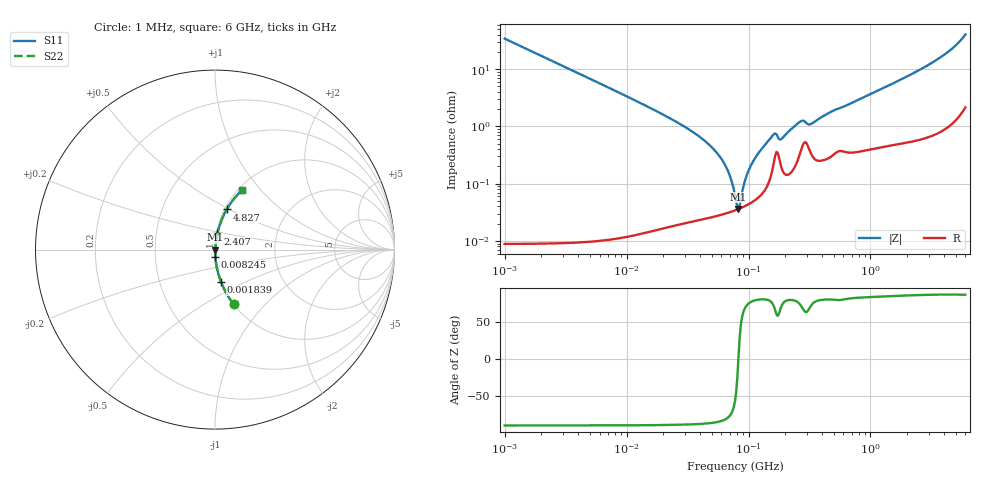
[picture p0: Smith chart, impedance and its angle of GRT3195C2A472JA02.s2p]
!Murata Part Number: GRT3195C2A472JA02
!These Parameters are Measured in Series Mode Connection
!Data Generated on Jun 19, 2026
!  o--ll--o
!Port1  Port2
!  o------o
!Operation Temp=25[degC], DC Bias Voltage=0[V]
!Freq. Start=1000[kHz] Stop=6[GHz] 401[Steps]
# Hz S RI R 50
!Freq.(Hz) S11(Real) S11(Imag) S21(Real) S21(Imag) S12(Real) S12(Imag) S22(Real) S22(Imag)
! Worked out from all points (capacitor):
!   401 points, 1 MHz to 6 GHz, reference 50 ohm
!   read as one part in series: C = 4.67 nF near 1.044 MHz
!   lowest |Z| = 36 mohm at 82.68 MHz (marker M1)
!   series resonance near 82.55 MHz, so ESL is about 800 pH
!   S11 on the Smith chart (normalised r, x): 1 MHz: 1.00, -0.68; 1.839 MHz: 1.00, -0.37; 8.245 MHz: 1.00, -0.08; 2.407 GHz: 1.01, +0.18; 4.827 GHz: 1.02, +0.48; 6 GHz: 1.04, +0.80
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1000000  0.104 -0.3052  0.896 0.3052  0.896 0.3052  0.104 -0.3052
1838529  0.0332 -0.179  0.9668 0.179  0.9668 0.179  0.0332 -0.179
4293785  0.00631 -0.0786  0.9937 0.0786  0.9937 0.0786  0.00631 -0.0786
8245209  0.00178 -0.0408  0.9982 0.0408  0.9982 0.0408  0.00178 -0.0408
1.843659e7  0.000464 -0.0175  0.9995 0.0175  0.9995 0.0175  0.000464 -0.0175
3.540316e7  0.00028 -0.00782  0.9997 0.00782  0.9997 0.00782  0.00028 -0.00782
5.236714e7  0.00028 -0.00388  0.9997 0.00388  0.9997 0.00388  0.00028 -0.00388
6.652088e7  0.000309 -0.0018  0.9997 0.0018  0.9997 0.0018  0.000309 -0.0018
7.256705e7  0.000325 -0.00107  0.9997 0.00107  0.9997 0.00107  0.000325 -0.00107
7.745967e7  0.000341 -0.00053  0.9997 0.00053  0.9997 0.00053  0.000341 -0.00053
8.268215e7  0.00036 1.34e-05  0.9996 -1.34e-05  0.9996 -1.34e-05  0.00036 1.34e-05
8.635799e7  0.000374 0.000377  0.9996 -0.000377  0.9996 -0.000377  0.000374 0.000377
9.627852e7  0.000419 0.0013  0.9996 -0.0013  0.9996 -0.0013  0.000419 0.0013
1.050294e8  0.000467 0.00206  0.9995 -0.00206  0.9995 -0.00206  0.000467 0.00206
1.553559e8  0.00163 0.00648  0.9984 -0.00648  0.9984 -0.00648  0.00163 0.00648
1.848803e8  0.00204 0.00558  0.998 -0.00558  0.998 -0.00558  0.00204 0.00558
2.675853e8  0.00376 0.0116  0.9962 -0.0116  0.9962 -0.0116  0.00376 0.0116
3.325952e8  0.00316 0.0108  0.9968 -0.0108  0.9968 -0.0108  0.00316 0.0108
1.428092e9  0.00723 0.0516  0.9928 -0.0516  0.9928 -0.0516  0.00723 0.0516
2.40683e9  0.0138 0.0897  0.9862 -0.0897  0.9862 -0.0897  0.0138 0.0897
4.827224e9  0.0652 0.2236  0.9348 -0.2236  0.9348 -0.2236  0.0652 0.2236
6e9  0.152 0.3333  0.848 -0.3333  0.848 -0.3333  0.152 0.3333
